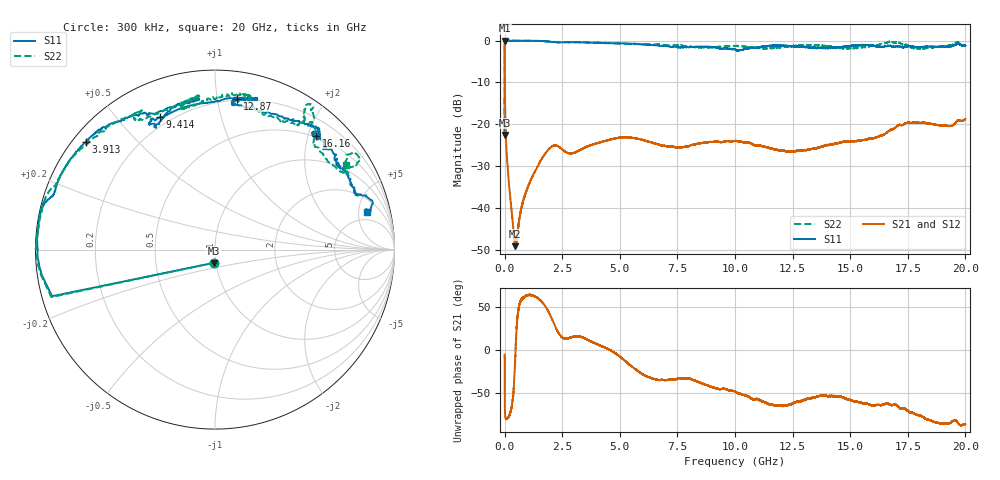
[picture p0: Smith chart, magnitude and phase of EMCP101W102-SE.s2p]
!EMCP101W102
!Johanson Technology Inc.
!www.johansontechnology.com
!Test Board Conditions:
!Substrate Type  RO4350B
!Substrate Thickness  10 mil
!Substrate Dk  3.66
!TL Type: GCPW
!TL Trace Width  20 mil
!TL Gap  10 mil
!PART MODE SINGLE ENDED (AKA BYPASS)
!DUT TOPOLOGY	SERIES-SHUNT
# MHz S  dB  R 50
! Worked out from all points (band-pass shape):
!   20001 points, 300 kHz to 20 GHz, reference 50 ohm
!   highest |S21| = -0.02 dB at 300 kHz (marker M1); lowest = -49.2 dB at 466.3 MHz (marker M2)
!   |S21| within 3 dB of the highest: start of sweep to 3.727 MHz
!   lowest |S11| = -22.6 dB at 300 kHz (marker M3), VSWR 1.16, Z = 48.9 - j7.26 ohm
!   |S11| at or under -10 dB: start of sweep to 1.288 MHz
!   |S22| runs from -22.7 to 0.0 dB; largest |S21 - S12| = 0.0035
!   S11 on the Smith chart (normalised r, x): 300 kHz: 0.98, -0.15; 3.913 GHz: 0.04, +0.36; 9.414 GHz: 0.16, +0.66; 12.87 GHz: 0.19, +1.14; 16.16 GHz: 0.47, +2.14; 20 GHz: 3.59, +6.25
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0.3  -22.60 -94.8  -0.01 -5.1  -0.00 -5.0  -22.69 -94.2
101.298  -0.10 -178.7  -28.08 -80.7  -28.08 -80.7  -0.06 -178.8
148.298  -0.12 -180.0  -31.65 -79.5  -31.68 -79.2  -0.01 179.8
363.295  -0.08 176.2  -44.09 -54.5  -44.26 -55.7  -0.04 177.1
466.293  -0.08 174.9  -49.16 -6.4  -48.92 -5.5  -0.05 176.0
943.286  -0.07 169.4  -36.02 63.5  -35.94 63.5  -0.08 171.1
1801.273  -0.21 163.9  -26.74 50.1  -26.74 50.2  -0.16 161.2
3334.25  -0.44 148.5  -25.99 15.4  -25.97 15.4  -0.42 152.1
3913.241  -0.56 140.2  -24.70 8.2  -24.70 8.1  -0.47 147.8
5258.221  -0.67 132.7  -23.13 -13.2  -23.10 -13.2  -0.85 135.6
6667.2  -1.20 120.6  -24.81 -35.0  -24.79 -35.5  -0.97 126.1
8341.175  -1.51 96.5  -24.73 -36.7  -24.75 -36.7  -1.58 118.3
9414.159  -1.97 112.5  -24.29 -45.7  -24.17 -45.5  -1.46 99.1
10000.15  -2.13 116.4  -23.99 -48.6  -23.98 -48.5  -1.33 96.5
11657.12  -1.21 76.3  -25.92 -64.2  -25.88 -64.2  -1.77 98.9
12871.11  -1.41 81.7  -26.38 -59.8  -26.38 -59.9  -1.19 80.7
13334.1  -1.77 83.4  -25.95 -56.0  -25.83 -55.5  -1.16 77.8
15118.07  -1.26 53.1  -24.04 -59.9  -24.02 -60.5  -1.80 64.5
16163.06  -1.41 48.3  -23.07 -64.4  -23.07 -64.3  -1.11 55.3
16667.05  -1.28 49.1  -21.62 -63.2  -21.76 -61.4  -0.33 57.4
18500.02  -1.43 28.8  -19.95 -82.7  -19.85 -83.2  -1.71 32.3
20000  -1.19 13.8  -18.74 -87.2  -18.68 -88.7  -1.22 32.6
